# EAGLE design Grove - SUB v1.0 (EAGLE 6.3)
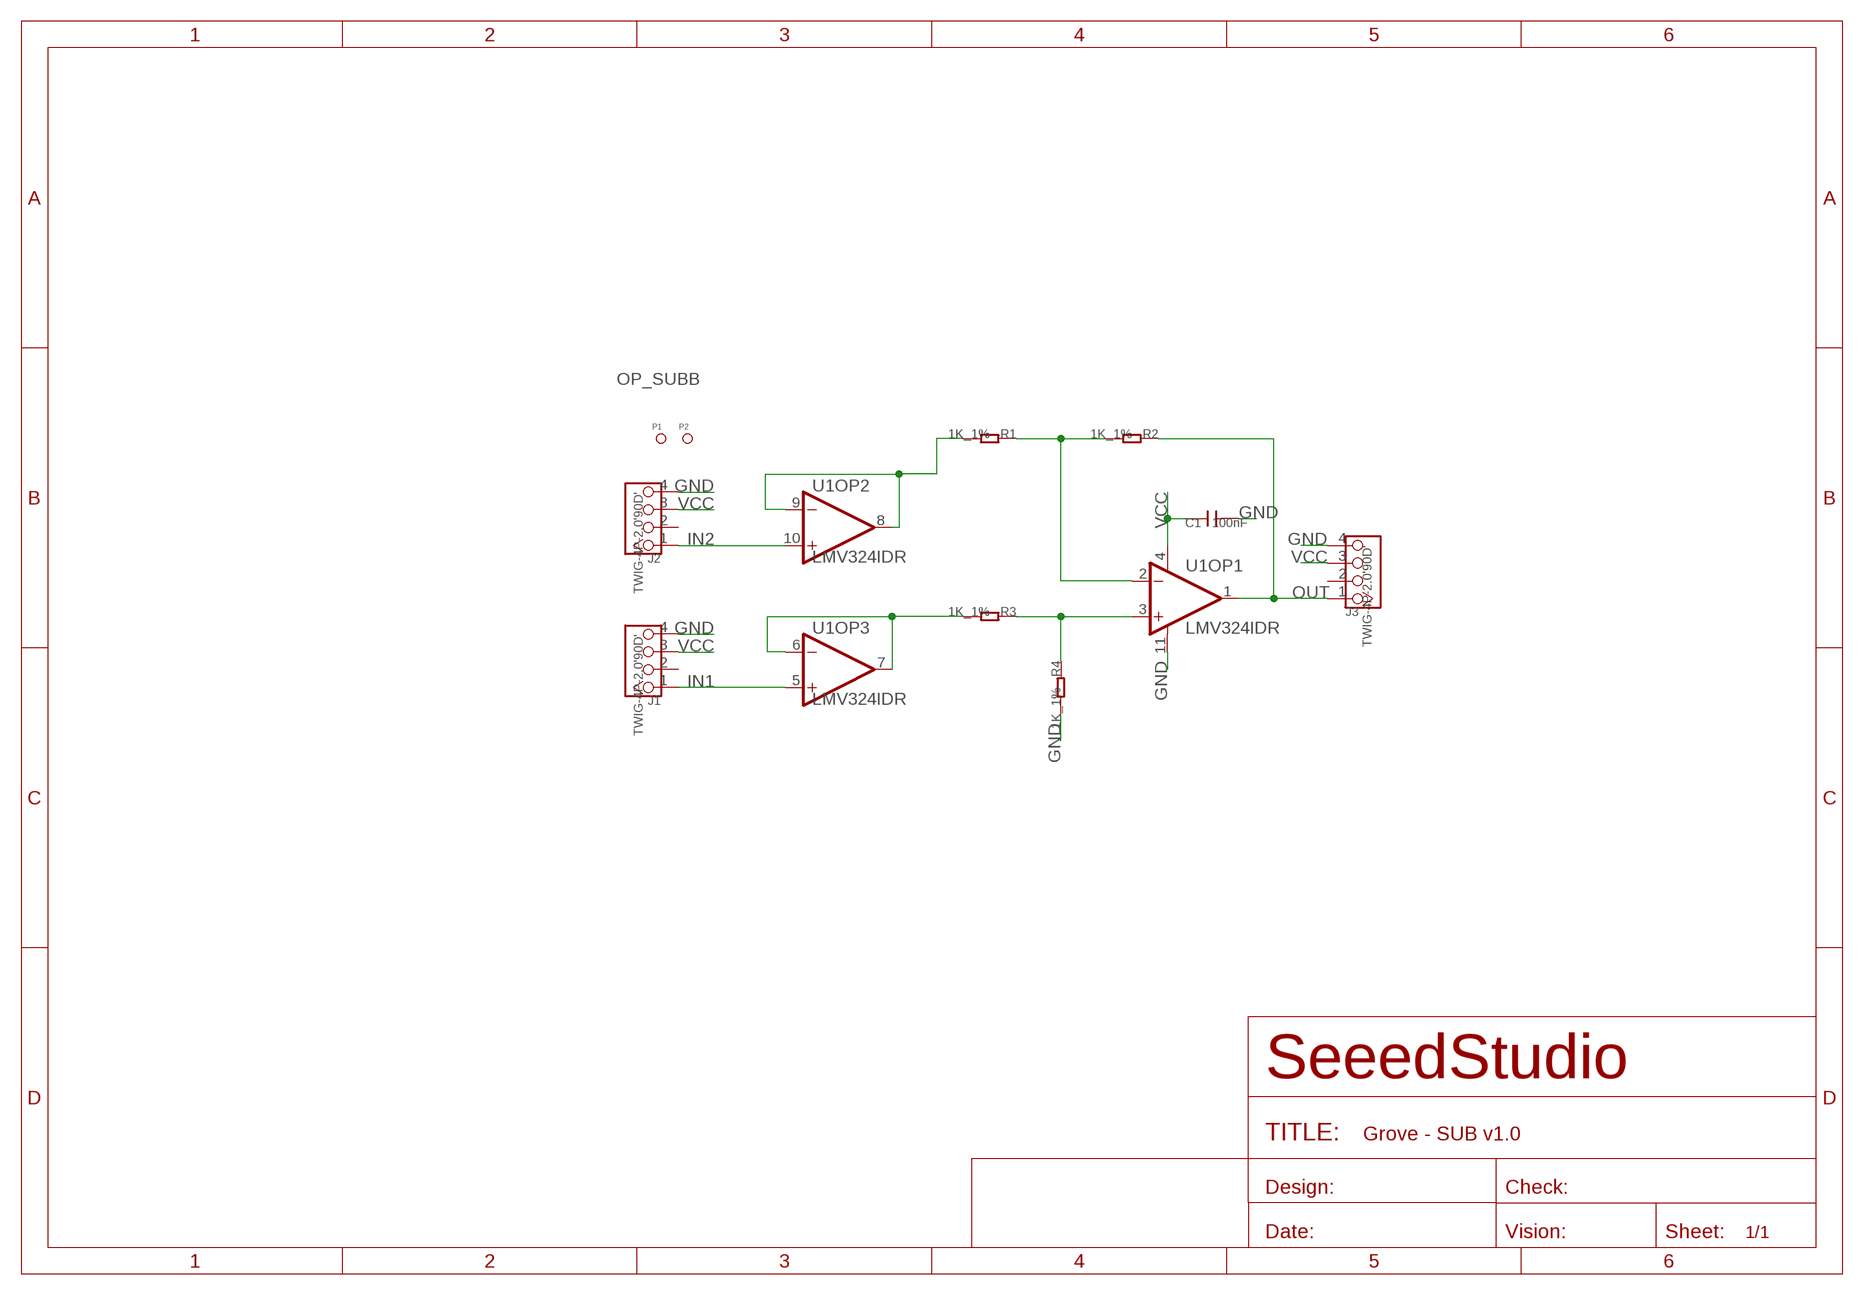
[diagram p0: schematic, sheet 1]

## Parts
C1  100nF  C-0603  [C0603]
J1  TWIG-4P-2.0'90D'  [4P-2.0-90D]
J2  TWIG-4P-2.0'90D'  [4P-2.0-90D]
J3  TWIG-4P-2.0'90D'  [4P-2.0-90D]
P1  PAD-MARK  [ROUND-MARK-1.0]
P2  PAD-MARK  [ROUND-MARK-1.0]
R1  1K_1%  R-0603  [R0603]
R2  1K_1%  R-0603  [R0603]
R3  1K_1%  R-0603  [R0603]
R4  1K_1%  R-0603  [R0603]
U1  LMV324IDR  LMV324-SO014  [SO014]

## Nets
GND: C1.2 J1.4 J2.4 J3.4 R4.2 U1.11(OP1:V-)
IN1: J1.1 U1.5(OP3:IN+)
IN2: J2.1 U1.10(OP2:IN+)
N$23: R3.1 R4.1 U1.3(OP1:IN+)
N$24: R1.1 R2.2 U1.2(OP1:IN-)
N$31: R3.2 U1.6(OP3:IN-) U1.7(OP3:OUT)
N$32: R1.2 U1.8(OP2:OUT) U1.9(OP2:IN-)
OUT: J3.1 R2.1 U1.1(OP1:OUT)
VCC: C1.1 J1.3 J2.3 J3.3 U1.4(OP1:V+)
Unconnected: J1.2 J2.2 J3.2 U1.12(OP4:IN+) U1.13(OP4:IN-) U1.14(OP4:OUT)

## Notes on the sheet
- OP_SUBB

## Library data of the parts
C1 = Discrete:C*: Ceramic Capacitors
J1-J3 = Connector:TWIG-4P-2.0
P1 P2 = Discrete:PAD-MARK; PARTNO: DNP
R1-R4 = Discrete:R*
U1 = IC:LMV324: General purpose LOW Voltage, Rail-to-Rail Output Amplifiers http://www.fairchildsemi.com/ds/LM/LMV358.pdf

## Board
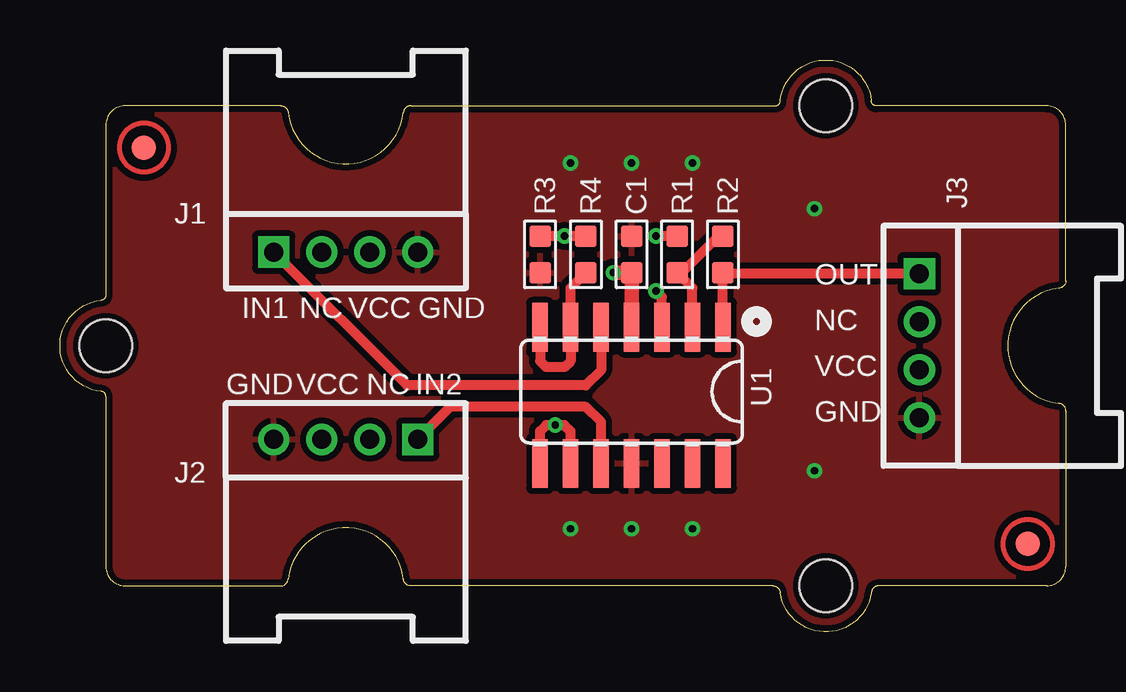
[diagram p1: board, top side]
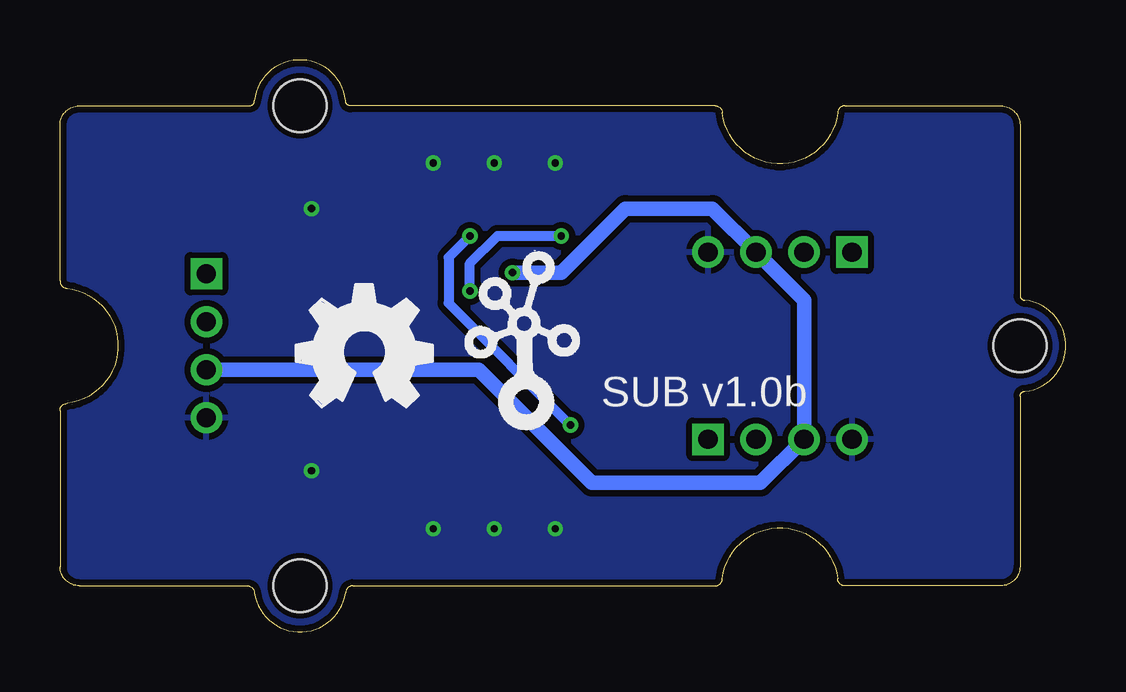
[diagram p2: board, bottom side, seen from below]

Size 41.91 x 23.83 mm. Coordinates in mm from the lower left corner, seen from the top.
Copper layers (1*16): Top 0.035mm / dielectric 1.5mm / Bottom 0.035mm
Design rules "SeeedStudio_rule_no_angle_090911": minimum track width 6mil, minimum drill 12mil, track to track 6mil, track to pad 6mil, pad to pad 6mil, via to via 6mil, smd to smd 0mil, copper to edge 10mil, drill to drill 10mil, minimum pad ring 10mil, minimum via ring 6mil, stop-mask expansion 2mil, vias tented up to drill 100mil, thermal gap 10mil

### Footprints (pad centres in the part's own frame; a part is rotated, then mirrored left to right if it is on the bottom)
C0603 = smd 0.889 x 0.889: 1 -0.762,0; 2 0.762,0
4P-2.0-90D = drill 0.8 pad 1.27 square: 1 -3,0 | drill 0.8 pad 1.27: 2 -1,0; 3 1,0; 4 3,0
ROUND-MARK-1.0 = smd 1.016 x 1.016: P$1 0,0
R0603 = smd 0.889 x 0.889: 1 -0.762,0; 2 0.762,0
SO014 = smd 0.66 x 2.032: 1 -3.175,-2.68; 2 -1.905,-2.68; 3 -0.635,-2.68; 4 0.635,-2.68; 5 1.905,-2.68; 6 3.175,-2.68; 7 4.445,-2.68; 8 4.445,2.997; 9 3.175,2.997; 10 1.905,2.997; 11 0.635,2.997; 12 -0.635,2.997; 13 -1.905,2.997; 14 -3.175,2.997
2U-DIM-W/DRILL = hole 2.2: -10,-10; -10,10; 20,0

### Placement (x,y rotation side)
C1  23.81,15.73 90 top
J1  11.91,15.82 0 top
J2  11.91,8.02 180 top
J3  35.81,11.92 270 top
P1  3.49,20.18 0 top
P2  40.32,3.67 0 top
R1  25.72,15.73 90 top
R2  27.62,15.73 90 top
R3  21.91,15.73 270 top
R4  20,15.73 270 top
U1  24.45,10.02 180 top
U$2  [2U-DIM-W/DRILL]  21.91,11.92 180 top
U$3  [OSHW_FILLX200_NOTEXT]  32.07,9.38 0 bottom
U$4  [TWIGLOGO]  22.54,9.38 0 bottom

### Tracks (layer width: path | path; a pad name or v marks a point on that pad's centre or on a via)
GND  (via drill 0.3 pad 0.64)
  other vias: 26.35,19.54 21.27,4.3 23.81,4.3 26.35,4.3 31.43,17.64 31.43,6.71 21.27,19.54 23.81,19.54
  pour Top (isolate 0.254): -0.32,-0.14 42.23,-0.14 42.23,23.99 -0.32,23.99
  pour Bottom (isolate 0.254): -0.32,-0.14 42.23,-0.14 42.23,23.99 -0.32,23.99
IN1
  Top 0.406: U1.5 22.54,10.91 21.91,10.27 14.46,10.27 J1.1
IN2
  Top 0.406: U1.10 22.54,8.75 21.91,9.38 16.27,9.38 J2.1
N$23  (via drill 0.3 pad 0.64)
  Top 0.406: R3.1 v21.02,16.49 R4.1 | U1.3 25.08,13.95 v24.83,14.21
  Bottom 0.406: v21.02,16.49 23.69,16.49 24.83,15.35 v24.83,14.21
N$24
  Top 0.406: U1.2 26.35,14.33 R1.1 25.91,14.97 27.43,16.49 R2.2
N$31
  Top 0.406: R3.2 21.27,14.33 U1.6 21.27,11.29 21.02,11.03 20.26,11.03 20,11.29 U1.7
N$32  (via drill 0.3 pad 0.64)
  Top 0.406: U1.9 21.27,8.37 21.02,8.62 v20.64,8.62 20.26,8.62 20,8.37 U1.8 | R1.2 v24.83,16.49
  Bottom 0.406: v24.83,16.49 25.72,15.6 25.72,13.7 v20.64,8.62
OUT
  Top 0.406: U1.1 R2.1 27.67,14.92 J3.1
VCC  (via drill 0.3 pad 0.64)
  Top 0.61: U1.4 C1.1 v23.05,14.97
  Bottom 0.61: J3.3 24.46,10.92 19.75,6.21 12.72,6.21 J2.3 10.91,13.82 J1.3 14.72,17.64 18.35,17.64 21.02,14.97 v23.05,14.97

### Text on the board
tPlace: OUT | IN1 | NC | VCC | GND | NC | VCC | GND | VCC | NC | IN2 | GND
bPlace: SUB v1.0b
